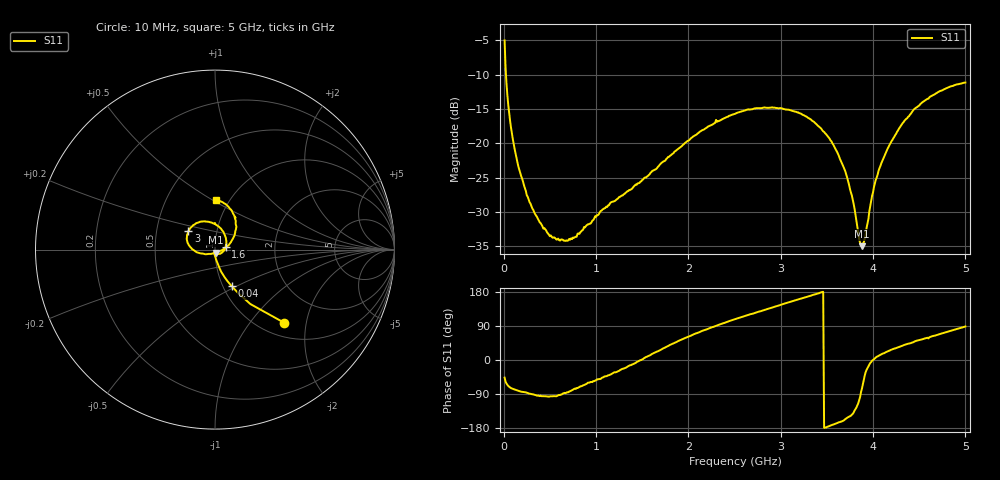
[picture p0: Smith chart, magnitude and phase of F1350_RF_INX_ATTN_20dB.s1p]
! S-parameters for RF_INX input IDT F1350 DPD Demodulator
! Date Measured:  2015-11-25  RGG
!  Port 1 = Pin 35 = RF_INX
! STATE: RF_INX selected, 20 dB attenuation (Gain = Gmax - 20 dB)
! RF Frequency:  10 MHz to 5000 MHz
! RF_INY, IF_I+, IF_I-, IF_Q+, and IF_Q- terminated
! 2300 MHz, 0 dBm signal applied to LO_IN
! Vcc = +5.00 Volts  Icc = approx 275 mA.
! NOTES:  The device was measured on a custom printed circuit evaluation board with individual 50 ohm
!  microstrip lines to the RF and LO pins. The 50 ohm microstrip lines were de-embedded using reference
!  plane extensions
! Instrument Manufacturer:  Agilent Technologies
! Instrument Model:  E5071C
! Instrument Serial Number:  MY46419053
! Instrument Firmware Rev:  A.11.31
! Frequency Re{S11} Im{S11}
# HZ  S  RI R 50.00
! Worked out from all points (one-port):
!   500 points, 10 MHz to 5 GHz, reference 50 ohm
!   lowest |S11| = -35.0 dB at 3.88 GHz (marker M1), VSWR 1.04, Z = 50.4 - j1.73 ohm
!   |S11| at or under -10 dB: 24.9 MHz to end of sweep
!   S11 on the Smith chart (normalised r, x): 10 MHz: 1.26, -1.51; 40 MHz: 1.10, -0.47; 1.6 GHz: 1.13, +0.04; 3 GHz: 0.73, +0.15; 5 GHz: 0.87, +0.52
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1e7  0.387 -0.4084
4e7  0.0928 -0.2037
8e7  0.035 -0.1242
1.3e8  0.0163 -0.0816
2.7e8  0.00125 -0.0389
4.8e8  -0.0024 -0.0218
6.4e8  0.000466 -0.0198
7.7e8  0.00518 -0.0199
1.26e9  0.0364 -0.0182
1.6e9  0.0595 0.0162
1.89e9  0.0584 0.0696
2.14e9  0.0305 0.1198
2.51e9  -0.0513 0.1563
3e9  -0.1491 0.1017
3.13e9  -0.1565 0.0712
3.34e9  -0.1443 0.0226
3.53e9  -0.1072 -0.0114
3.68e9  -0.0632 -0.023
3.76e9  -0.0367 -0.0238
3.85e9  -0.00521 -0.0193
3.88e9  0.00455 -0.0172
3.92e9  0.0183 -0.0114
4.01e9  0.048 0.00185
4.08e9  0.0664 0.0164
4.2e9  0.092 0.0475
4.38e9  0.1142 0.1064
4.63e9  0.1045 0.1945
5e9  0.00741 0.2773
